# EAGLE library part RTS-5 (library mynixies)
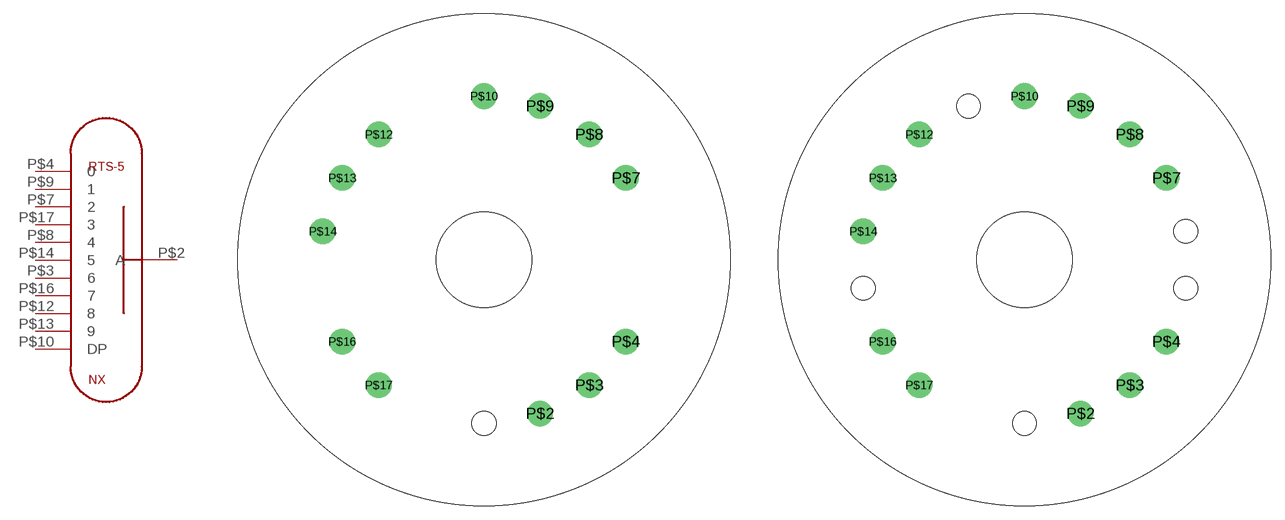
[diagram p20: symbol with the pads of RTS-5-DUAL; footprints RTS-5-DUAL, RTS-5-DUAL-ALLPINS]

Designator prefix NX

## RTS-5  [RTS-5-DUAL]
P$2  A  pas
P$3  6  pas
P$4  0  pas
P$7  2  pas
P$8  4  pas
P$9  1  pas
P$10  DP  pas
P$12  8  pas
P$13  9  pas
P$14  5  pas
P$16  7  pas
P$17  3  pas

## RTS-5ALLPINS  [RTS-5-DUAL-ALLPINS]
Pads as for RTS-5-DUAL

## RTS-5NL8091  [RTS-5-TOP-VIEW]
P$2  A  pas
P$3  0  pas
P$4  9  pas
P$7  8  pas
P$8  7  pas
P$9  6  pas
P$10  DP  pas
P$12  5  pas
P$13  4  pas
P$14  3  pas
P$16  2  pas
P$17  1  pas

## Footprint RTS-5-DUAL (pad centres in mm)
drill 1.829: P$2 5.973,-16.409; P$3 11.225,-13.377; P$4 15.123,-8.731; P$7 15.123,8.731; P$8 11.225,13.377; P$9 5.973,16.409; P$10 0,17.462; P$12 -11.225,13.377; P$13 -15.123,8.731; P$14 -17.197,3.032; P$16 -15.123,-8.731; P$17 -11.225,-13.377
hole 10.16 at 0,0

## Footprint RTS-5-DUAL-ALLPINS (pad centres in mm)
drill 1.829: P$2 5.973,-16.409; P$3 11.225,-13.377; P$4 15.123,-8.731; P$7 15.123,8.731; P$8 11.225,13.377; P$9 5.973,16.409; P$10 0,17.462; P$12 -11.225,13.377; P$13 -15.123,8.731; P$14 -17.197,3.032; P$16 -15.123,-8.731; P$17 -11.225,-13.377
hole 10.16 at 0,0
hole 2.54 at 0,-17.462
hole 2.54 at 17.197,-3.032
hole 2.54 at 17.197,3.032
hole 2.54 at -5.973,16.409
hole 2.54 at -17.197,-3.032

## Footprint RTS-5-TOP-VIEW (pad centres in mm)
drill 1.829: P$2 5.973,-16.409; P$3 11.225,-13.377; P$4 15.123,-8.731; P$7 15.123,8.731; P$8 11.225,13.377; P$9 5.973,16.409; P$10 0,17.462; P$12 -11.225,13.377; P$13 -15.123,8.731; P$14 -17.197,3.032; P$16 -15.123,-8.731; P$17 -11.225,-13.377
hole 10.16 at 0,0
hole 2.54 at 0,-17.462
hole 2.54 at 17.197,-3.032
hole 2.54 at 17.197,3.032
hole 2.54 at -5.973,16.409
hole 2.54 at -17.197,-3.032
